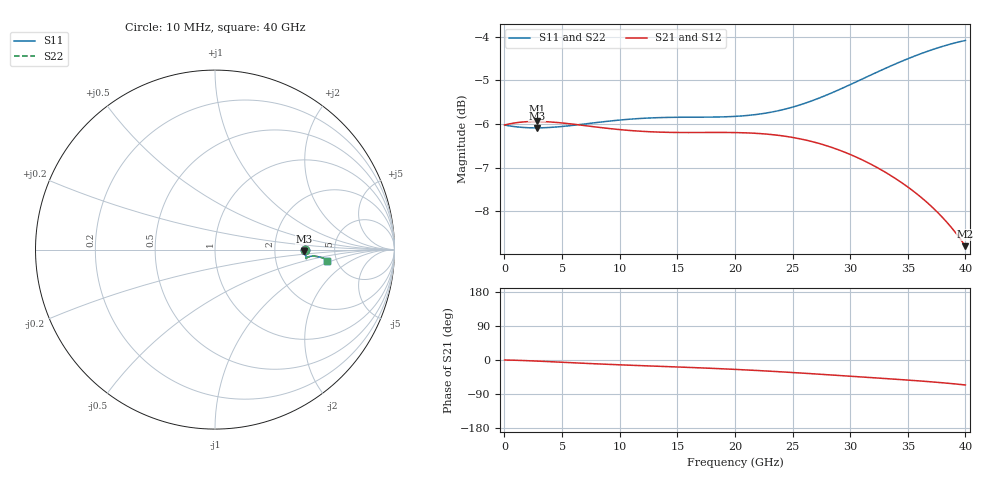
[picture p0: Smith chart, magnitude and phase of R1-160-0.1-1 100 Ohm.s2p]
!version-1
!date-09.2020
# MHz S RI R 50
!Freq ReS11 ImS11 ReS21 ImS21 ReS12 ImS12 ReS22 ImS22
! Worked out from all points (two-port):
!   101 points, 10 MHz to 40 GHz, reference 50 ohm
!   highest |S21| = -5.94 dB at 2.81 GHz (marker M1); lowest = -8.8 dB at 40 GHz (marker M2)
!   |S21| within 3 dB of the highest: start of sweep to end of sweep
!   lowest |S11| = -6.1 dB at 2.81 GHz (marker M3), VSWR 2.97, Z = 148 - j3.21 ohm
!   |S11| at or under -10 dB: nowhere
!   |S22| runs from -6.1 to -4.1 dB; largest |S21 - S12| = 0
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10  0.5 -2.7e-05  0.5 -4.92e-05  0.5 -4.92e-05  0.5 -2.7e-05
1210  0.4973 -0.00336  0.5034 -0.00846  0.5034 -0.00846  0.4973 -0.00336
2810  0.4962 -0.00816  0.5041 -0.0251  0.5041 -0.0251  0.4962 -0.00816
4410  0.4971 -0.0135  0.5016 -0.0446  0.5016 -0.0446  0.4971 -0.0135
6810  0.5006 -0.0226  0.494 -0.0741  0.494 -0.0741  0.5006 -0.0226
9610  0.5049 -0.0335  0.4834 -0.1047  0.4834 -0.1047  0.5049 -0.0335
11610  0.5069 -0.0404  0.4762 -0.124  0.4762 -0.124  0.5069 -0.0404
13610  0.5079 -0.0457  0.4696 -0.1423  0.4696 -0.1423  0.5079 -0.0457
16810  0.508 -0.0498  0.459 -0.172  0.459 -0.172  0.508 -0.0498
20010  0.5093 -0.0484  0.445 -0.2054  0.445 -0.2054  0.5093 -0.0484
22010  0.5124 -0.0454  0.4324 -0.2284  0.4324 -0.2284  0.5124 -0.0454
23610  0.517 -0.0425  0.4193 -0.2475  0.4193 -0.2475  0.517 -0.0425
25210  0.5236 -0.0398  0.4033 -0.2664  0.4033 -0.2664  0.5236 -0.0398
26810  0.5324 -0.0377  0.3845 -0.2843  0.3845 -0.2843  0.5324 -0.0377
28810  0.546 -0.0366  0.3573 -0.3043  0.3573 -0.3043  0.546 -0.0366
30410  0.5582 -0.0373  0.3331 -0.3175  0.3331 -0.3175  0.5582 -0.0373
32010  0.5709 -0.0391  0.3073 -0.3278  0.3073 -0.3278  0.5709 -0.0391
33610  0.5835 -0.0417  0.2802 -0.3352  0.2802 -0.3352  0.5835 -0.0417
35610  0.5981 -0.0458  0.244 -0.3403  0.244 -0.3403  0.5981 -0.0458
37210  0.6085 -0.0496  0.2124 -0.3408  0.2124 -0.3408  0.6085 -0.0496
38810  0.6171 -0.0548  0.1772 -0.3375  0.1772 -0.3375  0.6171 -0.0548
40000  0.622 -0.0607  0.148 -0.3317  0.148 -0.3317  0.622 -0.0607
